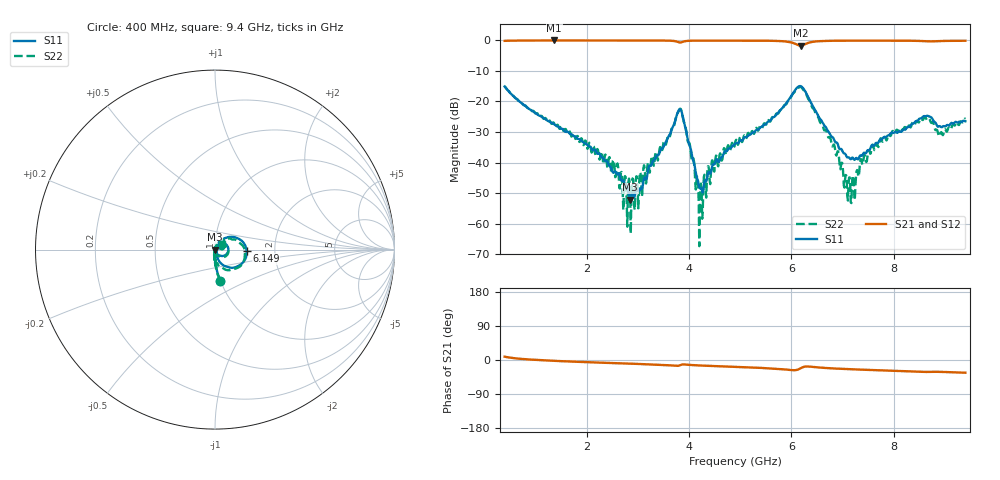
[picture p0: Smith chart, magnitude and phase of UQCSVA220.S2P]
!  Part Number  UQCSVA220  Mounting Orientation: Horizontal
!  Description: Ultra Low ESR Microwave capacitors
!  Application: Coupling, Bypass, Tuning, DC Block
!  Filters, Matching
# GHZ S DB R 50
! Freq  |S11|  S11 Ph  |S21|  S21 Ph  |S12|  S12 Ph  |S22|  S22 Ph
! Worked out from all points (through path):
!   801 points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, 400 MHz to 9.4 GHz, reference 50 ohm
!   highest |S21| = -0.03 dB at 1.368 GHz (marker M1); lowest = -1.7 dB at 6.183 GHz (marker M2)
!   group delay of S21, straight-line fit = 11 ps
!   lowest |S11| = -52.2 dB at 2.853 GHz (marker M3), VSWR 1.00, Z = 49.8 - j0.0848 ohm
!   |S11| at or under -10 dB: start of sweep to end of sweep
!   |S22| runs from -67.4 to -15.0 dB; largest |S21 - S12| = 0.015
!   S11 on the Smith chart (normalised r, x): 400 MHz: 0.99, -0.36; 6.149 GHz: 1.43, -0.02; 9.4 GHz: 1.07, +0.07
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0.4  -15.09 -80.8  -0.16 8.7  -0.09 8.7  -14.99 -80.6
1.368  -27.47 -92.1  -0.03 -2.2  -0.01 -2.4  -27.18 -94.3
1.908  -33.08 -96.2  -0.03 -5.2  -0.01 -5.4  -32.16 -95.8
2.56  -42.92 -104.9  -0.05 -8.3  -0.01 -8.5  -44.81 -92.1
2.751  -47.25 -133.6  -0.04 -9.2  -0.01 -9.4  -44.44 -52.5
2.853  -52.19 -159.7  -0.04 -9.7  -0.01 -9.9  -50.53 -75.5
2.976  -48.90 152.9  -0.04 -10.2  -0.01 -10.5  -44.49 7.2
3.404  -37.57 72.0  -0.06 -12.4  0.00 -12.8  -38.61 67.8
3.831  -22.57 -5.1  -0.71 -13.5  -0.66 -13.8  -22.36 -12.8
4.236  -48.32 -15.7  -0.07 -14.6  -0.03 -15.0  -46.89 -18.0
4.495  -40.62 54.1  -0.07 -16.0  -0.03 -16.4  -42.96 64.7
4.9  -33.98 63.3  -0.07 -18.0  -0.04 -18.5  -33.74 69.9
6.149  -15.05 -2.0  -1.64 -24.2  -1.64 -24.7  -15.41 -11.8
6.183  -14.99 -14.1  -1.71 -21.7  -1.70 -22.3  -15.25 -23.9
6.408  -21.18 -65.4  -0.51 -18.1  -0.51 -18.6  -21.97 -79.1
6.88  -33.46 -61.9  -0.12 -22.7  -0.14 -23.3  -37.74 -93.6
7.139  -38.58 -28.3  -0.10 -24.2  -0.12 -24.8  -44.86 -36.9
7.386  -37.66 17.6  -0.09 -25.6  -0.12 -26.2  -40.74 42.3
7.904  -31.04 41.8  -0.09 -28.0  -0.13 -28.7  -30.71 46.1
8.624  -24.84 35.1  -0.27 -31.5  -0.32 -32.2  -25.30 20.2
8.916  -28.25 27.4  -0.22 -31.3  -0.28 -32.0  -30.20 23.1
9.4  -26.50 44.3  -0.13 -33.6  -0.20 -34.3  -25.74 38.5
